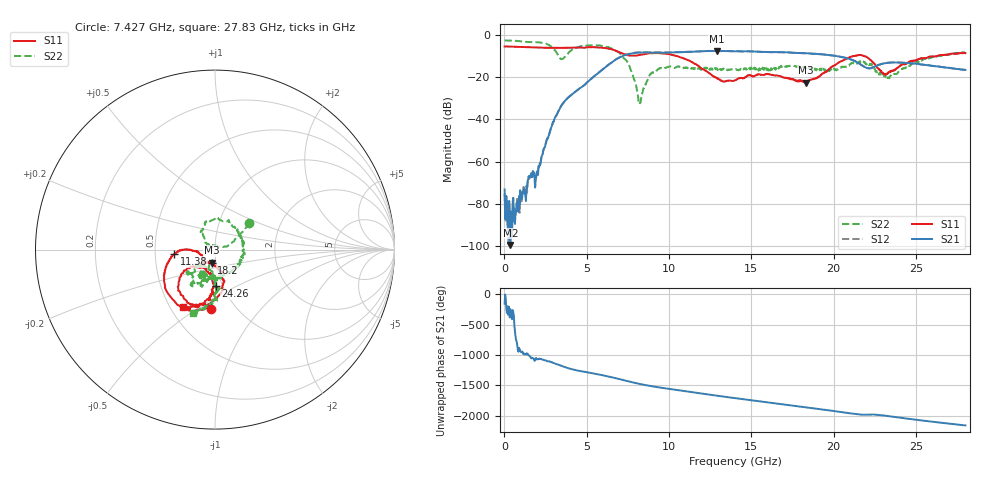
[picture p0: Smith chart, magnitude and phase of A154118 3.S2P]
!  2-Port S-parameters saved by WinCal
! VAR MeasName=S-Parameters (CALIBRATED_DATA) read from VNA (N5230A)
! VAR MeasDate=2015-9-10 14:34:42
! VAR NAME=A154118 3
! VAR FILENAME=A154118 3.S2P
! VAR DATE=2015-9-10 14:34:42
! VAR PHYS_PORTS=1,2
# Hz S DB R 50
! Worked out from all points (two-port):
!   801 points, 10 MHz to 28 GHz, reference 50 ohm
!   highest |S21| = -7.64 dB at 12.89 GHz (marker M1); lowest = -99.4 dB at 359.9 MHz (marker M2)
!   |S21| within 3 dB of the highest: 7.012 GHz to 20.57 GHz (13.55 GHz wide, 98.3 % of centre)
!   lowest |S11| = -22.6 dB at 18.31 GHz (marker M3), VSWR 1.16, Z = 47.8 - j6.93 ohm
!   |S11| at or under -10 dB: 10.44 GHz to 21.24 GHz (10.79 GHz wide, 68.1 % of centre); 21.27624 GHz to 21.32056 GHz (44.32 MHz wide, 0.208 % of centre); 21.8 GHz to 26.3 GHz (4.504 GHz wide, 18.7 % of centre)
!   |S22| runs from -32.8 to -2.7 dB; largest |S21 - S12| = 0.0076
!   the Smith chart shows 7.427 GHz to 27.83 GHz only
!   S11 on the Smith chart (normalised r, x): 7.427 GHz: 0.77, -0.57; 11.38 GHz: 0.63, -0.03; 18.2 GHz: 0.95, -0.14; 24.26 GHz: 0.93, -0.39; 27.83 GHz: 0.58, -0.43
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1e7  -5.53 179.6  -73.09 -157.5  -75.01 -121.4  -2.67 179.8
3.59875e8  -5.55 168.0  -99.38 115.3  -85.60 -19.1  -2.72 171.1
1.9693e9  -6.02 116.8  -64.59 14.0  -65.06 17.2  -3.47 129.1
3.193862e9  -6.12 72.3  -37.53 -71.0  -37.53 -70.7  -8.71 25.6
3.753662e9  -6.11 49.6  -30.54 -125.9  -30.54 -125.7  -9.83 -108.7
4.698325e9  -6.10 8.5  -24.66 171.3  -24.64 171.5  -5.33 166.6
6.202788e9  -6.38 -57.3  -14.88 94.2  -14.80 94.1  -5.71 100.6
7.42735e9  -9.57 -94.2  -9.35 14.6  -9.31 14.3  -12.40 37.8
8.232062e9  -9.50 -99.9  -8.39 -35.6  -8.31 -35.9  -32.23 97.3
9.351662e9  -8.65 -126.0  -8.47 -90.5  -8.38 -90.7  -16.05 111.7
1.138094e10  -12.88 -174.1  -8.03 -170.3  -7.99 -171.0  -15.72 27.4
1.28854e10  -20.34 -170.9  -7.64 132.9  -7.61 132.2  -15.84 -38.0
1.4005e10  -21.50 -136.1  -7.79 92.2  -7.79 91.7  -16.45 -72.6
1.620921e10  -18.90 -130.7  -8.20 15.7  -8.20 15.0  -15.74 -97.0
1.82035e10  -22.44 -104.7  -8.66 -53.9  -8.69 -54.4  -15.62 -114.1
1.830846e10  -22.60 -103.4  -8.70 -58.0  -8.67 -57.9  -15.86 -115.1
1.869332e10  -21.07 -92.1  -8.88 -71.2  -8.91 -71.8  -15.25 -117.1
2.152731e10  -9.63 -113.2  -13.50 -176.3  -13.38 -177.0  -13.20 -122.0
2.334666e10  -17.81 -107.2  -13.19 155.6  -13.13 154.7  -20.47 -108.8
2.425634e10  -13.81 -89.1  -13.21 122.7  -13.24 122.0  -15.88 -90.2
2.782506e10  -8.69 -118.9  -16.44 8.2  -16.48 6.8  -8.57 -109.1
2.8e10  -8.67 -120.4  -16.57 3.0  -16.63 1.9  -8.07 -112.3
